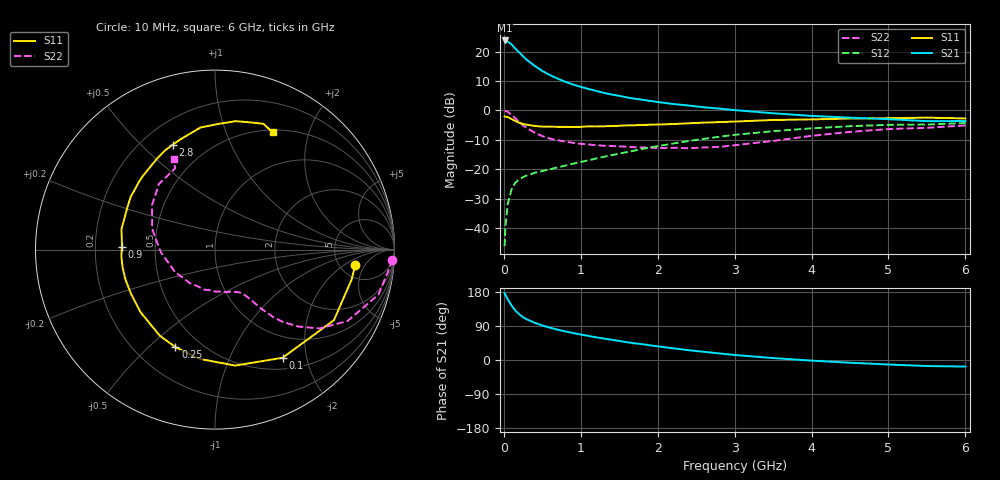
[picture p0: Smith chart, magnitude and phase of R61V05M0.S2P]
! SIEMENS Small Signal Semiconductors
! BFR193
! Si NPN RF Bipolar Junction Transistor in SOT23
! VCE = 1 V  IC = 5 mA
! Common Emitter S-Parameters:  May  1996
# GHz  S  MA  R  50
!  f  S11  S21  S12  S22
! GHz  MAG  ANG  MAG  ANG  MAG  ANG  MAG  ANG
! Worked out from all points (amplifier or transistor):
!   36 points, 10 MHz to 6 GHz, reference 50 ohm
!   highest |S21| = 23.8 dB at 10 MHz (marker M1)
!   |S21| within 3 dB of that: start of sweep to 158.7 MHz
!   unconditionally stable (mu >= 1): 868 MHz to 2.196 GHz
!   at 250 MHz: K = 0.44, MSG = 20.5 dB, |S12| = -22.7 dB
!   at 1.4 GHz: K = 1.08, MAG = 8.6 dB, |S12| = -15.3 dB
!   at 6 GHz: K = 0.99, MSG = 0.3 dB, |S12| = -4.3 dB
!   S11 on the Smith chart (normalised r, x): 10 MHz: 6.93, -3.14; 100 MHz: 0.66, -1.60; 250 MHz: 0.37, -0.61; 900 MHz: 0.32, +0.01; 2.8 GHz: 0.32, +0.63; 6 GHz: 0.53, +1.47
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0.01  0.7867 -6.3  15.42 176.3  0.0049 86.4  0.9886 -3.2
0.02  0.7789 -12.5  15.11 172.0  0.0103 85.1  0.9763 -6.3
0.05  0.7706 -30.7  14.78 160.6  0.0255 74.2  0.9444 -15.4
0.1  0.7105 -58.0  13.21 143.9  0.0452 63.0  0.8391 -28.3
0.15  0.656 -80.1  11.2 130.6  0.0587 54.8  0.7298 -37.0
0.2  0.6147 -98.4  9.67 120.6  0.0671 49.8  0.6322 -42.7
0.25  0.5863 -112.1  8.299 112.9  0.0732 46.6  0.5526 -46.8
0.3  0.5699 -122.7  7.19 107.2  0.0782 45.0  0.4974 -49.2
0.4  0.5419 -140.0  5.715 98.3  0.0864 43.8  0.4186 -51.9
0.5  0.5289 -152.3  4.674 91.0  0.0927 44.5  0.3634 -53.7
0.6  0.526 -161.5  3.973 85.2  0.0997 45.7  0.3308 -55.0
0.7  0.5245 -169.1  3.456 80.0  0.1073 47.2  0.3103 -56.3
0.9  0.5194 178.1  2.745 71.2  0.1238 49.9  0.2798 -59.4
1.1  0.5336 167.6  2.308 63.5  0.1415 52.4  0.2623 -64.3
1.3  0.5355 158.9  1.984 56.6  0.1621 53.8  0.2496 -69.6
1.6  0.5547 147.7  1.654 46.9  0.195 54.4  0.2402 -79.7
2.2  0.5842 128.6  1.281 30.9  0.2721 51.6  0.2311 -105.3
2.8  0.6307 111.9  1.071 17.4  0.3555 44.5  0.2387 -139.5
3.5  0.6849 96.8  0.891 5.1  0.4421 33.5  0.3016 -177.1
4.5  0.7247 80.9  0.75 -7.2  0.5372 17.2  0.4297 144.7
5.5  0.7511 68.9  0.654 -15.9  0.5734 1.4  0.5041 116.2
6  0.7282 63.9  0.658 -17.3  0.6076 -3.3  0.5534 114.5
